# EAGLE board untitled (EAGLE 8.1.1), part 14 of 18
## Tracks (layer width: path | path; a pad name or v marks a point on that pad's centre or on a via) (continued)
S$14098 (continued)
  Bottom 0: 231.52,137.75 231.07,137.79
S$14099
  Bottom 0: 231.07,137.79 230.63,137.75
S$14100
  Bottom 0: 230.63,137.75 230.2,137.62
S$14101
  Bottom 0: 230.2,137.62 229.8,137.41
S$14102
  Bottom 0: 229.8,137.41 229.46,137.12
S$14103
  Bottom 0: 229.46,137.12 229.17,136.78
S$14104
  Bottom 0: 229.17,136.78 228.96,136.38
S$14105
  Bottom 0: 228.96,136.38 228.83,135.96
S$14106
  Bottom 0: 228.83,135.96 228.79,135.51
S$14107
  Bottom 0: 228.79,135.51 228.83,135.06
S$14108
  Bottom 0: 228.83,135.06 228.96,134.63
S$14109
  Bottom 0: 228.96,134.63 229.17,134.24
S$14110
  Bottom 0: 229.17,134.24 229.46,133.89
S$14111
  Bottom 0: 229.46,133.89 229.8,133.61
S$14112
  Bottom 0: 229.8,133.61 230.16,133.42
S$14113
  Bottom 0: 230.16,133.42 225.02,133.42
S$14114
  Bottom 0: 225.02,133.42 215.78,142.65
S$14115
  Bottom 0: 215.78,142.65 216.1,142.67
S$14116
  Bottom 0: 216.1,142.67 216.4,142.78
S$14117
  Bottom 0: 216.4,142.78 216.67,142.97
S$14118
  Bottom 0: 216.67,142.97 216.87,143.22
S$14119
  Bottom 0: 216.87,143.22 217,143.52
S$14120
  Bottom 0: 217,143.52 217.05,143.84
S$14121
  Bottom 0: 217.05,143.84 217,144.16
S$14122
  Bottom 0: 217,144.16 216.87,144.46
S$14123
  Bottom 0: 216.87,144.46 216.67,144.71
S$14124
  Bottom 0: 216.67,144.71 216.4,144.9
S$14125
  Bottom 0: 216.4,144.9 216.1,145.01
S$14126
  Bottom 0: 216.1,145.01 215.77,145.03
S$14127
  Bottom 0: 215.77,145.03 215.45,144.96
S$14128
  Bottom 0: 215.45,144.96 215.16,144.82
S$14129
  Bottom 0: 215.16,144.82 214.93,144.59
S$14130
  Bottom 0: 214.93,144.59 214.76,144.32
S$14131
  Bottom 0: 214.76,144.32 214.67,144
S$14132
  Bottom 0: 214.67,144 214.67,143.77
S$14133
  Bottom 0: 214.67,143.77 199.64,158.8
S$14134
  Bottom 0: 199.64,158.8 199.64,158.84
S$14135
  Bottom 0: 199.64,158.84 199.63,158.91
S$14136
  Bottom 0: 199.63,158.91 199.62,158.98
S$14137
  Bottom 0: 199.62,158.98 199.59,159.04
S$14138
  Bottom 0: 199.59,159.04 199.55,159.1
S$14139
  Bottom 0: 199.55,159.1 199.51,159.16
S$14140
  Bottom 0: 199.51,159.16 198.6,160.06
S$14141
  Bottom 0: 198.6,160.06 198.55,160.1
S$14142
  Bottom 0: 198.55,160.1 198.49,160.14
S$14143
  Bottom 0: 198.49,160.14 198.43,160.17
S$14144
  Bottom 0: 198.43,160.17 198.36,160.18
S$14145
  Bottom 0: 198.36,160.18 198.29,160.19
S$14146
  Bottom 0: 198.29,160.19 197.07,160.19
S$14147
  Bottom 0: 197.07,160.19 197,160.18
S$14148
  Bottom 0: 197,160.18 196.93,160.17
S$14149
  Bottom 0: 196.93,160.17 196.87,160.14
S$14150
  Bottom 0: 196.87,160.14 196.81,160.1
S$14151
  Bottom 0: 196.81,160.1 196.76,160.06
S$14152
  Bottom 0: 196.76,160.06 191.71,155.01
S$14153
  Bottom 0: 191.71,155.01 191.67,154.95
S$14154
  Bottom 0: 191.67,154.95 191.63,154.89
S$14155
  Bottom 0: 191.63,154.89 191.6,154.83
S$14156
  Bottom 0: 191.6,154.83 191.59,154.76
S$14157
  Bottom 0: 191.59,154.76 191.58,154.7
S$14158
  Bottom 0: 191.58,154.7 191.58,153.34
S$14159
  Bottom 0: 191.58,153.34 191.43,153.28
S$14160
  Bottom 0: 191.43,153.28 191.13,153.1
S$14161
  Bottom 0: 191.13,153.1 190.9,152.84
S$14162
  Bottom 0: 190.9,152.84 190.76,152.6
S$14163
  Bottom 0: 190.76,152.6 189.38,152.6
S$14164
  Bottom 0: 189.38,152.6 189.48,152.66
S$14165
  Bottom 0: 189.48,152.66 189.83,152.94
S$14166
  Bottom 0: 189.83,152.94 190.11,153.29
S$14167
  Bottom 0: 190.11,153.29 190.33,153.68
S$14168
  Bottom 0: 190.33,153.68 190.45,154.11
S$14169
  Bottom 0: 190.45,154.11 190.5,154.56
S$14170
  Bottom 0: 190.5,154.56 190.45,155.01
S$14171
  Bottom 0: 190.45,155.01 190.33,155.43
S$14172
  Bottom 0: 190.33,155.43 190.11,155.83
S$14173
  Bottom 0: 190.11,155.83 189.83,156.17
S$14174
  Bottom 0: 189.83,156.17 189.48,156.46
S$14175
  Bottom 0: 189.48,156.46 189.09,156.67
S$14176
  Bottom 0: 189.09,156.67 188.66,156.8
S$14177
  Bottom 0: 188.66,156.8 188.21,156.84
S$14178
  Bottom 0: 188.21,156.84 187.77,156.8
S$14179
  Bottom 0: 187.77,156.8 187.34,156.67
S$14180
  Bottom 0: 187.34,156.67 186.94,156.46
S$14181
  Bottom 0: 186.94,156.46 186.6,156.17
S$14182
  Bottom 0: 186.6,156.17 186.31,155.83
S$14183
  Bottom 0: 186.31,155.83 186.1,155.43
S$14184
  Bottom 0: 186.1,155.43 185.97,155.01
S$14185
  Bottom 0: 185.97,155.01 185.93,154.56
S$14186
  Bottom 0: 185.93,154.56 185.97,154.11
S$14187
  Bottom 0: 185.97,154.11 186.1,153.68
S$14188
  Bottom 0: 186.1,153.68 186.31,153.29
S$14189
  Bottom 0: 186.31,153.29 186.6,152.94
S$14190
  Bottom 0: 186.6,152.94 186.94,152.66
S$14191
  Bottom 0: 186.94,152.66 187.05,152.6
S$14192
  Bottom 0: 187.05,152.6 177.17,152.6
S$14193
  Bottom 0: 177.17,152.6 175.9,153.88
S$14194
  Bottom 0: 175.9,153.88 175.84,153.92
S$14195
  Bottom 0: 175.84,153.92 175.78,153.96
S$14196
  Bottom 0: 175.78,153.96 175.72,153.99
S$14197
  Bottom 0: 175.72,153.99 175.65,154
S$14198
  Bottom 0: 175.65,154 175.58,154
S$14199
  Bottom 0: 175.58,154 171.91,154
S$14200
  Bottom 0: 171.91,154 171.84,154
S$14201
  Bottom 0: 171.84,154 171.77,153.99
S$14202
  Bottom 0: 171.77,153.99 171.71,153.96
S$14203
  Bottom 0: 171.71,153.96 171.65,153.92
S$14204
  Bottom 0: 171.65,153.92 171.59,153.88
S$14205
  Bottom 0: 171.59,153.88 171.13,153.42
S$14206
  Bottom 0: 171.13,153.42 171.28,153.68
S$14207
  Bottom 0: 171.28,153.68 171.4,154.11
S$14208
  Bottom 0: 171.4,154.11 171.45,154.56
S$14209
  Bottom 0: 171.45,154.56 171.4,155.01
S$14210
  Bottom 0: 171.4,155.01 171.28,155.43
S$14211
  Bottom 0: 171.28,155.43 171.06,155.83
S$14212
  Bottom 0: 171.06,155.83 170.78,156.17
S$14213
  Bottom 0: 170.78,156.17 170.43,156.46
S$14214
  Bottom 0: 170.43,156.46 170.04,156.67
S$14215
  Bottom 0: 170.04,156.67 169.61,156.8
S$14216
  Bottom 0: 169.61,156.8 169.16,156.84
S$14217
  Bottom 0: 169.16,156.84 168.72,156.8
S$14218
  Bottom 0: 168.72,156.8 168.29,156.67
S$14219
  Bottom 0: 168.29,156.67 167.89,156.46
S$14220
  Bottom 0: 167.89,156.46 167.55,156.17
S$14221
  Bottom 0: 167.55,156.17 167.26,155.83
S$14222
  Bottom 0: 167.26,155.83 167.05,155.43
S$14223
  Bottom 0: 167.05,155.43 166.92,155.01
S$14224
  Bottom 0: 166.92,155.01 166.88,154.56
S$14225
  Bottom 0: 166.88,154.56 166.92,154.11
S$14226
  Bottom 0: 166.92,154.11 167.05,153.68
S$14227
  Bottom 0: 167.05,153.68 167.26,153.29
S$14228
  Bottom 0: 167.26,153.29 167.55,152.94
S$14229
  Bottom 0: 167.55,152.94 167.89,152.66
S$14230
  Bottom 0: 167.89,152.66 168.08,152.56
S$14231
  Bottom 0: 168.08,152.56 158.57,152.56
S$14232
  Bottom 0: 158.57,152.56 158.57,156.7
S$14233
  Bottom 0: 158.57,156.7 158.56,156.77
S$14234
  Bottom 0: 158.56,156.77 158.55,156.84
S$14235
  Bottom 0: 158.55,156.84 158.52,156.9
S$14236
  Bottom 0: 158.52,156.9 158.48,156.96
S$14237
  Bottom 0: 158.48,156.96 158.44,157.02
S$14238
  Bottom 0: 158.44,157.02 153.73,161.73
S$14239
  Bottom 0: 153.73,161.73 153.86,161.71
S$14240
  Bottom 0: 153.86,161.71 154.18,161.73
S$14241
  Bottom 0: 154.18,161.73 154.49,161.83
S$14242
  Bottom 0: 154.49,161.83 154.75,162.02
S$14243
  Bottom 0: 154.75,162.02 154.96,162.28
S$14244
  Bottom 0: 154.96,162.28 155.09,162.57
S$14245
  Bottom 0: 155.09,162.57 155.13,162.89
S$14246
  Bottom 0: 155.13,162.89 155.09,163.22
S$14247
  Bottom 0: 155.09,163.22 154.96,163.51
S$14248
  Bottom 0: 154.96,163.51 154.75,163.77
S$14249
  Bottom 0: 154.75,163.77 154.49,163.96
S$14250
  Bottom 0: 154.49,163.96 154.18,164.06
S$14251
  Bottom 0: 154.18,164.06 153.86,164.08
S$14252
  Bottom 0: 153.86,164.08 153.54,164.02
S$14253
  Bottom 0: 153.54,164.02 153.25,163.87
S$14254
  Bottom 0: 153.25,163.87 153.01,163.65
S$14255
  Bottom 0: 153.01,163.65 152.84,163.37
S$14256
  Bottom 0: 152.84,163.37 152.76,163.06
S$14257
  Bottom 0: 152.76,163.06 152.76,162.73
S$14258
  Bottom 0: 152.76,162.73 152.77,162.69
S$14259
  Bottom 0: 152.77,162.69 145.38,170.08
S$14260
  Bottom 0: 145.38,170.08 145.41,170.11
S$14261
  Bottom 0: 145.41,170.11 145.62,170.4
S$14262
  Bottom 0: 145.62,170.4 145.75,170.72
S$14263
  Bottom 0: 145.75,170.72 145.8,171.07
S$14264
  Bottom 0: 145.8,171.07 145.75,171.41
S$14265
  Bottom 0: 145.75,171.41 145.62,171.74
S$14266
  Bottom 0: 145.62,171.74 145.41,172.02
S$14267
  Bottom 0: 145.41,172.02 145.15,172.25
S$14268
  Bottom 0: 145.15,172.25 144.83,172.4
S$14269
  Bottom 0: 144.83,172.4 144.49,172.46
S$14270
  Bottom 0: 144.49,172.46 144.13,172.44
S$14271
  Bottom 0: 144.13,172.44 143.81,172.33
S$14272
  Bottom 0: 143.81,172.33 143.51,172.15
S$14273
  Bottom 0: 143.51,172.15 143.27,171.89
S$14274
  Bottom 0: 143.27,171.89 143.1,171.58
S$14275
  Bottom 0: 143.1,171.58 143.01,171.24
S$14276
  Bottom 0: 143.01,171.24 143.01,170.9
S$14277
  Bottom 0: 143.01,170.9 143.1,170.56
S$14278
  Bottom 0: 143.1,170.56 143.27,170.25
S$14279
  Bottom 0: 143.27,170.25 143.51,169.99
S$14280
  Bottom 0: 143.51,169.99 143.81,169.8
S$14281
  Bottom 0: 143.81,169.8 144.13,169.7
S$14282
  Bottom 0: 144.13,169.7 144.49,169.68
S$14283
  Bottom 0: 144.49,169.68 144.52,169.68
S$14284
  Bottom 0: 144.52,169.68 147.18,167.02
S$14285
  Bottom 0: 147.18,167.02 142.66,167.02
S$14286
  Bottom 0: 142.66,167.02 138.47,171.23
S$14287
  Bottom 0: 138.47,171.23 138.47,171.28
S$14288
  Bottom 0: 138.47,171.28 138.43,171.53
S$14289
  Bottom 0: 138.43,171.53 138.3,171.74
S$14290
  Bottom 0: 138.3,171.74 138.09,171.89
S$14291
  Bottom 0: 138.09,171.89 137.85,171.96
S$14292
  Bottom 0: 137.85,171.96 137.6,171.94
S$14293
  Bottom 0: 137.6,171.94 137.38,171.83
S$14294
  Bottom 0: 137.38,171.83 137.2,171.64
S$14295
  Bottom 0: 137.2,171.64 137.11,171.4
S$14296
  Bottom 0: 137.11,171.4 137.11,171.15
S$14297
  Bottom 0: 137.11,171.15 137.2,170.92
S$14298
  Bottom 0: 137.2,170.92 137.38,170.73
S$14299
  Bottom 0: 137.38,170.73 137.6,170.62
S$14300
  Bottom 0: 137.6,170.62 137.85,170.6
S$14301
  Bottom 0: 137.85,170.6 138.67,169.76
S$14302
  Bottom 0: 138.67,169.76 138.48,169.86
S$14303
  Bottom 0: 138.48,169.86 138.13,169.92
S$14304
  Bottom 0: 138.13,169.92 137.78,169.9
S$14305
  Bottom 0: 137.78,169.9 137.46,169.79
S$14306
  Bottom 0: 137.46,169.79 137.16,169.61
S$14307
  Bottom 0: 137.16,169.61 136.92,169.35
S$14308
  Bottom 0: 136.92,169.35 136.8,169.14
S$14309
  Bottom 0: 136.8,169.14 136.8,174.28
S$14310
  Bottom 0: 136.8,174.28 139.63,177.1
S$14311
  Bottom 0: 139.63,177.1 139.66,177.16
S$14312
  Bottom 0: 139.66,177.16 139.7,177.2
S$14313
  Bottom 0: 139.7,177.2 139.71,177.25
S$14314
  Bottom 0: 139.71,177.25 139.74,177.3
S$14315
  Bottom 0: 139.74,177.3 139.74,177.36
S$14316
  Bottom 0: 139.74,177.36 139.76,177.42
S$14317
  Bottom 0: 139.76,177.42 139.76,177.55
S$14318
  Bottom 0: 139.76,177.55 140.21,177.55
S$14319
  Bottom 0: 140.21,177.55 140.28,177.56
S$14320
  Bottom 0: 140.28,177.56 140.35,177.6
S$14321
  Bottom 0: 140.35,177.6 140.41,177.65
S$14322
  Bottom 0: 140.41,177.65 140.45,177.72
S$14323
  Bottom 0: 140.45,177.72 140.46,177.8
S$14324
  Bottom 0: 140.46,177.8 140.46,179.51
S$14325
  Bottom 0: 140.46,179.51 141.07,179.51
S$14326
  Bottom 0: 141.07,179.51 140.9,179.31
S$14327
  Bottom 0: 140.9,179.31 140.76,179.01
S$14328
  Bottom 0: 140.76,179.01 140.72,178.69
S$14329
  Bottom 0: 140.72,178.69 140.76,178.37
S$14330
  Bottom 0: 140.76,178.37 140.9,178.07
S$14331
  Bottom 0: 140.9,178.07 141.11,177.82
S$14332
  Bottom 0: 141.11,177.82 141.39,177.65
S$14333
  Bottom 0: 141.39,177.65 141.7,177.56
S$14334
  Bottom 0: 141.7,177.56 142.02,177.56
S$14335
  Bottom 0: 142.02,177.56 142.33,177.65
S$14336
  Bottom 0: 142.33,177.65 142.61,177.82
S$14337
  Bottom 0: 142.61,177.82 142.82,178.07
S$14338
  Bottom 0: 142.82,178.07 142.96,178.37
S$14339
  Bottom 0: 142.96,178.37 143,178.69
S$14340
  Bottom 0: 143,178.69 142.96,179.01
S$14341
  Bottom 0: 142.96,179.01 142.82,179.31
S$14342
  Bottom 0: 142.82,179.31 142.65,179.51
S$14343
  Bottom 0: 142.65,179.51 157.23,179.51
S$14344
  Bottom 0: 157.23,179.51 157.23,177.8
S$14345
  Bottom 0: 157.23,177.8 157.24,177.72
S$14346
  Bottom 0: 157.24,177.72 157.28,177.65
S$14347
  Bottom 0: 157.28,177.65 157.33,177.6
S$14348
  Bottom 0: 157.33,177.6 157.4,177.56
S$14349
  Bottom 0: 157.4,177.56 157.48,177.55
S$14350
  Bottom 0: 157.48,177.55 157.87,177.55
S$14351
  Bottom 0: 157.87,177.55 155.15,174.83
S$14352
  Bottom 0: 155.15,174.83 155.1,174.77
S$14353
  Bottom 0: 155.1,174.77 155.07,174.72
S$14354
  Bottom 0: 155.07,174.72 155.04,174.65
S$14355
  Bottom 0: 155.04,174.65 155.02,174.58
S$14356
  Bottom 0: 155.02,174.58 155.01,174.51
S$14357
  Bottom 0: 155.01,174.51 155.01,166.12
S$14358
  Bottom 0: 155.01,166.12 154.92,166.03
S$14359
  Bottom 0: 154.92,166.03 154.75,165.75
S$14360
  Bottom 0: 154.75,165.75 154.66,165.43
S$14361
  Bottom 0: 154.66,165.43 154.66,165.11
S$14362
  Bottom 0: 154.66,165.11 154.75,164.79
S$14363
  Bottom 0: 154.75,164.79 154.92,164.52
S$14364
  Bottom 0: 154.92,164.52 155.15,164.3
S$14365
  Bottom 0: 155.15,164.3 155.44,164.15
S$14366
  Bottom 0: 155.44,164.15 155.76,164.08
S$14367
  Bottom 0: 155.76,164.08 156.09,164.1
S$14368
  Bottom 0: 156.09,164.1 156.39,164.21
S$14369
  Bottom 0: 156.39,164.21 156.66,164.4
S$14370
  Bottom 0: 156.66,164.4 156.87,164.65
S$14371
  Bottom 0: 156.87,164.65 156.99,164.95
S$14372
  Bottom 0: 156.99,164.95 157.04,165.27
S$14373
  Bottom 0: 157.04,165.27 156.99,165.59
S$14374
  Bottom 0: 156.99,165.59 156.87,165.89
S$14375
  Bottom 0: 156.87,165.89 156.66,166.15
S$14376
  Bottom 0: 156.66,166.15 156.39,166.33
S$14377
  Bottom 0: 156.39,166.33 156.09,166.44
S$14378
  Bottom 0: 156.09,166.44 155.9,166.45
S$14379
  Bottom 0: 155.9,166.45 155.9,167.83
S$14380
  Bottom 0: 155.9,167.83 155.97,167.71
S$14381
  Bottom 0: 155.97,167.71 156.21,167.45
S$14382
  Bottom 0: 156.21,167.45 156.5,167.26
S$14383
  Bottom 0: 156.5,167.26 156.84,167.16
S$14384
  Bottom 0: 156.84,167.16 157.19,167.14
S$14385
  Bottom 0: 157.19,167.14 157.53,167.2
S$14386
  Bottom 0: 157.53,167.2 157.85,167.35
S$14387
  Bottom 0: 157.85,167.35 158.12,167.57
S$14388
  Bottom 0: 158.12,167.57 158.32,167.86
S$14389
  Bottom 0: 158.32,167.86 158.45,168.18
S$14390
  Bottom 0: 158.45,168.18 158.5,168.53
S$14391
  Bottom 0: 158.5,168.53 158.45,168.87
S$14392
  Bottom 0: 158.45,168.87 158.32,169.2
S$14393
  Bottom 0: 158.32,169.2 158.12,169.48
S$14394
  Bottom 0: 158.12,169.48 157.85,169.71
S$14395
  Bottom 0: 157.85,169.71 157.53,169.86
S$14396
  Bottom 0: 157.53,169.86 157.19,169.92
S$14397
  Bottom 0: 157.19,169.92 156.84,169.9
S$14398
  Bottom 0: 156.84,169.9 156.5,169.79
S$14399
  Bottom 0: 156.5,169.79 156.21,169.61
S$14400
  Bottom 0: 156.21,169.61 155.97,169.35
S$14401
  Bottom 0: 155.97,169.35 155.9,169.22
S$14402
  Bottom 0: 155.9,169.22 155.9,174.33
S$14403
  Bottom 0: 155.9,174.33 158.68,177.1
S$14404
  Bottom 0: 158.68,177.1 158.71,177.16
S$14405
  Bottom 0: 158.71,177.16 158.75,177.2
S$14406
  Bottom 0: 158.75,177.2 158.76,177.25
S$14407
  Bottom 0: 158.76,177.25 158.79,177.3
S$14408
  Bottom 0: 158.79,177.3 158.79,177.36
S$14409
  Bottom 0: 158.79,177.36 158.81,177.42
S$14410
  Bottom 0: 158.81,177.42 158.81,177.55
S$14411
  Bottom 0: 158.81,177.55 159.26,177.55
S$14412
  Bottom 0: 159.26,177.55 159.33,177.56
S$14413
  Bottom 0: 159.33,177.56 159.41,177.6
S$14414
  Bottom 0: 159.41,177.6 159.46,177.65
S$14415
  Bottom 0: 159.46,177.65 159.5,177.72
S$14416
  Bottom 0: 159.5,177.72 159.51,177.8
S$14417
  Bottom 0: 159.51,177.8 159.51,179.51
S$14418
  Bottom 0: 159.51,179.51 160.12,179.51
S$14419
  Bottom 0: 160.12,179.51 159.95,179.31
S$14420
  Bottom 0: 159.95,179.31 159.81,179.01
S$14421
  Bottom 0: 159.81,179.01 159.77,178.69
S$14422
  Bottom 0: 159.77,178.69 159.81,178.37
S$14423
  Bottom 0: 159.81,178.37 159.95,178.07
S$14424
  Bottom 0: 159.95,178.07 160.16,177.82
S$14425
  Bottom 0: 160.16,177.82 160.44,177.65
S$14426
  Bottom 0: 160.44,177.65 160.75,177.56
S$14427
  Bottom 0: 160.75,177.56 161.07,177.56
S$14428
  Bottom 0: 161.07,177.56 161.2,177.6
S$14429
  Bottom 0: 161.2,177.6 161.59,177.2
S$14430
  Bottom 0: 161.59,177.2 161.59,174.78
S$14431
  Bottom 0: 161.59,174.78 161.54,174.88
S$14432
  Bottom 0: 161.54,174.88 161.25,175.22
S$14433
  Bottom 0: 161.25,175.22 160.91,175.51
S$14434
  Bottom 0: 160.91,175.51 160.51,175.72
S$14435
  Bottom 0: 160.51,175.72 160.09,175.85
S$14436
  Bottom 0: 160.09,175.85 159.64,175.9
S$14437
  Bottom 0: 159.64,175.9 159.19,175.85
S$14438
  Bottom 0: 159.19,175.85 158.76,175.72
S$14439
  Bottom 0: 158.76,175.72 158.37,175.51
S$14440
  Bottom 0: 158.37,175.51 158.02,175.22
S$14441
  Bottom 0: 158.02,175.22 157.74,174.88
S$14442
  Bottom 0: 157.74,174.88 157.52,174.48
S$14443
  Bottom 0: 157.52,174.48 157.4,174.06
S$14444
  Bottom 0: 157.4,174.06 157.35,173.61
S$14445
  Bottom 0: 157.35,173.61 157.4,173.16
S$14446
  Bottom 0: 157.4,173.16 157.52,172.74
S$14447
  Bottom 0: 157.52,172.74 157.74,172.34
S$14448
  Bottom 0: 157.74,172.34 158.02,171.99
S$14449
  Bottom 0: 158.02,171.99 158.37,171.71
S$14450
  Bottom 0: 158.37,171.71 158.76,171.5
S$14451
  Bottom 0: 158.76,171.5 159.19,171.37
S$14452
  Bottom 0: 159.19,171.37 159.64,171.32
S$14453
  Bottom 0: 159.64,171.32 160.09,171.37
S$14454
  Bottom 0: 160.09,171.37 160.51,171.5
S$14455
  Bottom 0: 160.51,171.5 160.91,171.71
S$14456
  Bottom 0: 160.91,171.71 161.11,171.87
S$14457
  Bottom 0: 161.11,171.87 161.11,163.22
S$14458
  Bottom 0: 161.11,163.22 161.11,163.12
S$14459
  Bottom 0: 161.11,163.12 161.13,163.04
S$14460
  Bottom 0: 161.13,163.04 161.17,162.95
S$14461
  Bottom 0: 161.17,162.95 161.21,162.88
S$14462
  Bottom 0: 161.21,162.88 161.28,162.81
S$14463
  Bottom 0: 161.28,162.81 166.24,157.85
S$14464
  Bottom 0: 166.24,157.85 166.3,157.79
S$14465
  Bottom 0: 166.3,157.79 166.38,157.74
S$14466
  Bottom 0: 166.38,157.74 166.46,157.71
S$14467
  Bottom 0: 166.46,157.71 166.55,157.69
S$14468
  Bottom 0: 166.55,157.69 166.64,157.68
S$14469
  Bottom 0: 166.64,157.68 169.05,157.68
S$14470
  Bottom 0: 169.05,157.68 169.14,157.69
S$14471
  Bottom 0: 169.14,157.69 169.22,157.71
S$14472
  Bottom 0: 169.22,157.71 169.31,157.74
S$14473
  Bottom 0: 169.31,157.74 169.38,157.79
S$14474
  Bottom 0: 169.38,157.79 169.45,157.85
S$14475
  Bottom 0: 169.45,157.85 170.14,158.55
S$14476
  Bottom 0: 170.14,158.55 170.27,158.51
S$14477
  Bottom 0: 170.27,158.51 170.6,158.51
S$14478
  Bottom 0: 170.6,158.51 170.9,158.6
S$14479
  Bottom 0: 170.9,158.6 171.18,158.78
S$14480
  Bottom 0: 171.18,158.78 171.39,159.02
S$14481
  Bottom 0: 171.39,159.02 171.53,159.32
S$14482
  Bottom 0: 171.53,159.32 171.58,159.64
S$14483
  Bottom 0: 171.58,159.64 171.53,159.96
S$14484
  Bottom 0: 171.53,159.96 171.39,160.26
S$14485
  Bottom 0: 171.39,160.26 171.18,160.5
S$14486
  Bottom 0: 171.18,160.5 170.9,160.68
S$14487
  Bottom 0: 170.9,160.68 170.6,160.77
S$14488
  Bottom 0: 170.6,160.77 170.27,160.77
S$14489
  Bottom 0: 170.27,160.77 169.96,160.68
S$14490
  Bottom 0: 169.96,160.68 169.69,160.5
S$14491
  Bottom 0: 169.69,160.5 169.47,160.26
S$14492
  Bottom 0: 169.47,160.26 169.34,159.96
S$14493
  Bottom 0: 169.34,159.96 169.29,159.64
S$14494
  Bottom 0: 169.29,159.64 169.33,159.34
S$14495
  Bottom 0: 169.33,159.34 169.04,159.04
S$14496
  Bottom 0: 169.04,159.04 169.04,160.53
S$14497
  Bottom 0: 169.04,160.53 169.03,160.6
S$14498
  Bottom 0: 169.03,160.6 168.99,160.68
S$14499
  Bottom 0: 168.99,160.68 168.93,160.73
S$14500
  Bottom 0: 168.93,160.73 168.86,160.77
S$14501
  Bottom 0: 168.86,160.77 168.78,160.78
S$14502
  Bottom 0: 168.78,160.78 168.34,160.78
S$14503
  Bottom 0: 168.34,160.78 168.34,160.91
S$14504
  Bottom 0: 168.34,160.91 168.28,161.13
S$14505
  Bottom 0: 168.28,161.13 168.11,161.29
S$14506
  Bottom 0: 168.11,161.29 167.89,161.35
S$14507
  Bottom 0: 167.89,161.35 167.54,161.35
S$14508
  Bottom 0: 167.54,161.35 166.45,162.43
S$14509
  Bottom 0: 166.45,162.43 166.52,162.57
S$14510
  Bottom 0: 166.52,162.57 166.56,162.89
S$14511
  Bottom 0: 166.56,162.89 166.52,163.22
S$14512
  Bottom 0: 166.52,163.22 166.39,163.51
S$14513
  Bottom 0: 166.39,163.51 166.18,163.77
S$14514
  Bottom 0: 166.18,163.77 165.92,163.96
S$14515
  Bottom 0: 165.92,163.96 165.61,164.06
S$14516
  Bottom 0: 165.61,164.06 165.29,164.08
S$14517
  Bottom 0: 165.29,164.08 164.97,164.02
S$14518
  Bottom 0: 164.97,164.02 164.68,163.87
S$14519
  Bottom 0: 164.68,163.87 164.44,163.65
S$14520
  Bottom 0: 164.44,163.65 164.27,163.37
S$14521
  Bottom 0: 164.27,163.37 164.19,163.06
S$14522
  Bottom 0: 164.19,163.06 164.19,162.73
S$14523
  Bottom 0: 164.19,162.73 164.27,162.42
S$14524
  Bottom 0: 164.27,162.42 164.44,162.14
S$14525
  Bottom 0: 164.44,162.14 164.68,161.92
S$14526
  Bottom 0: 164.68,161.92 164.97,161.77
S$14527
  Bottom 0: 164.97,161.77 165.29,161.71
S$14528
  Bottom 0: 165.29,161.71 165.61,161.73
S$14529
  Bottom 0: 165.61,161.73 165.84,161.8
S$14530
  Bottom 0: 165.84,161.8 166.89,160.75
S$14531
  Bottom 0: 166.89,160.75 166.86,160.73
S$14532
  Bottom 0: 166.86,160.73 166.8,160.68
S$14533
  Bottom 0: 166.8,160.68 166.76,160.6
S$14534
  Bottom 0: 166.76,160.6 166.75,160.53
S$14535
  Bottom 0: 166.75,160.53 166.75,158.94
S$14536
  Bottom 0: 166.75,158.94 162.25,163.45
S$14537
  Bottom 0: 162.25,163.45 162.25,170.38
S$14538
  Bottom 0: 162.25,170.38 162.32,170.25
S$14539
  Bottom 0: 162.32,170.25 162.56,169.99
S$14540
  Bottom 0: 162.56,169.99 162.85,169.8
S$14541
  Bottom 0: 162.85,169.8 163.19,169.7
S$14542
  Bottom 0: 163.19,169.7 163.53,169.68
S$14543
  Bottom 0: 163.53,169.68 163.88,169.74
S$14544
  Bottom 0: 163.88,169.74 164.06,169.82
S$14545
  Bottom 0: 164.06,169.82 167.43,166.46
S$14546
  Bottom 0: 167.43,166.46 167.49,166.42
S$14547
  Bottom 0: 167.49,166.42 167.55,166.38
S$14548
  Bottom 0: 167.55,166.38 167.61,166.35
S$14549
  Bottom 0: 167.61,166.35 167.68,166.33
S$14550
  Bottom 0: 167.68,166.33 167.75,166.33
S$14551
  Bottom 0: 167.75,166.33 171.33,166.33
S$14552
  Bottom 0: 171.33,166.33 174.01,163.64
S$14553
  Bottom 0: 174.01,163.64 174.07,163.6
S$14554
  Bottom 0: 174.07,163.6 174.13,163.56
S$14555
  Bottom 0: 174.13,163.56 174.19,163.53
S$14556
  Bottom 0: 174.19,163.53 174.26,163.52
S$14557
  Bottom 0: 174.26,163.52 174.33,163.51
S$14558
  Bottom 0: 174.33,163.51 178.12,163.51
S$14559
  Bottom 0: 178.12,163.51 178.19,163.52
S$14560
  Bottom 0: 178.19,163.52 178.25,163.53
S$14561
  Bottom 0: 178.25,163.53 178.31,163.56
S$14562
  Bottom 0: 178.31,163.56 178.37,163.6
S$14563
  Bottom 0: 178.37,163.6 178.43,163.64
S$14564
  Bottom 0: 178.43,163.64 180.96,166.17
S$14565
  Bottom 0: 180.96,166.17 181.75,166.17
S$14566
  Bottom 0: 181.75,166.17 181.59,166.02
S$14567
  Bottom 0: 181.59,166.02 181.42,165.75
S$14568
  Bottom 0: 181.42,165.75 181.34,165.43
S$14569
  Bottom 0: 181.34,165.43 181.34,165.1
S$14570
  Bottom 0: 181.34,165.1 181.38,164.93
S$14571
  Bottom 0: 181.38,164.93 179.91,163.46
S$14572
  Bottom 0: 179.91,163.46 174.03,163.46
S$14573
  Bottom 0: 174.03,163.46 174.01,163.51
S$14574
  Bottom 0: 174.01,163.51 173.8,163.77
S$14575
  Bottom 0: 173.8,163.77 173.54,163.96
S$14576
  Bottom 0: 173.54,163.96 173.23,164.06
S$14577
  Bottom 0: 173.23,164.06 172.91,164.08
S$14578
  Bottom 0: 172.91,164.08 172.66,164.03
S$14579
  Bottom 0: 172.66,164.03 171.02,165.67
S$14580
  Bottom 0: 171.02,165.67 170.95,165.74
S$14581
  Bottom 0: 170.95,165.74 170.88,165.78
S$14582
  Bottom 0: 170.88,165.78 170.79,165.81
S$14583
  Bottom 0: 170.79,165.81 170.71,165.84
S$14584
  Bottom 0: 170.71,165.84 170.62,165.84
S$14585
  Bottom 0: 170.62,165.84 164.51,165.84
S$14586
  Bottom 0: 164.51,165.84 164.49,165.89
S$14587
  Bottom 0: 164.49,165.89 164.28,166.15
S$14588
  Bottom 0: 164.28,166.15 164.01,166.33
S$14589
  Bottom 0: 164.01,166.33 163.71,166.44
S$14590
  Bottom 0: 163.71,166.44 163.38,166.46
S$14591
  Bottom 0: 163.38,166.46 163.06,166.4
S$14592
  Bottom 0: 163.06,166.4 162.77,166.25
S$14593
  Bottom 0: 162.77,166.25 162.54,166.03
S$14594
  Bottom 0: 162.54,166.03 162.37,165.75
S$14595
  Bottom 0: 162.37,165.75 162.28,165.43
S$14596
  Bottom 0: 162.28,165.43 162.28,165.11
S$14597
  Bottom 0: 162.28,165.11 162.37,164.79
S$14598
  Bottom 0: 162.37,164.79 162.54,164.52
S$14599
  Bottom 0: 162.54,164.52 162.77,164.3
S$14600
  Bottom 0: 162.77,164.3 163.06,164.15
S$14601
  Bottom 0: 163.06,164.15 163.38,164.08
S$14602
  Bottom 0: 163.38,164.08 163.71,164.1
S$14603
  Bottom 0: 163.71,164.1 164.01,164.21
S$14604
  Bottom 0: 164.01,164.21 164.28,164.4
S$14605
  Bottom 0: 164.28,164.4 164.49,164.65
S$14606
  Bottom 0: 164.49,164.65 164.51,164.7
S$14607
  Bottom 0: 164.51,164.7 170.38,164.7
S$14608
  Bottom 0: 170.38,164.7 171.85,163.23
S$14609
  Bottom 0: 171.85,163.23 171.81,163.06
S$14610
  Bottom 0: 171.81,163.06 171.81,162.73
S$14611
  Bottom 0: 171.81,162.73 171.89,162.42
S$14612
  Bottom 0: 171.89,162.42 172.06,162.14
S$14613
  Bottom 0: 172.06,162.14 172.3,161.92
S$14614
  Bottom 0: 172.3,161.92 172.59,161.77
S$14615
  Bottom 0: 172.59,161.77 172.91,161.71
S$14616
  Bottom 0: 172.91,161.71 173.23,161.73
S$14617
  Bottom 0: 173.23,161.73 173.54,161.83
S$14618
  Bottom 0: 173.54,161.83 173.8,162.02
S$14619
  Bottom 0: 173.8,162.02 174.01,162.28
S$14620
  Bottom 0: 174.01,162.28 174.03,162.33
S$14621
  Bottom 0: 174.03,162.33 180.15,162.33
S$14622
  Bottom 0: 180.15,162.33 180.24,162.33
S$14623
  Bottom 0: 180.24,162.33 180.32,162.35
S$14624
  Bottom 0: 180.32,162.35 180.41,162.38
S$14625
  Bottom 0: 180.41,162.38 180.48,162.43
S$14626
  Bottom 0: 180.48,162.43 180.55,162.49
S$14627
  Bottom 0: 180.55,162.49 182.18,164.13
S$14628
  Bottom 0: 182.18,164.13 182.44,164.08
S$14629
  Bottom 0: 182.44,164.08 182.76,164.1
S$14630
  Bottom 0: 182.76,164.1 183.07,164.21
S$14631
  Bottom 0: 183.07,164.21 183.33,164.39
S$14632
  Bottom 0: 183.33,164.39 183.54,164.65
S$14633
  Bottom 0: 183.54,164.65 183.56,164.7
S$14634
  Bottom 0: 183.56,164.7 189.44,164.7
S$14635
  Bottom 0: 189.44,164.7 190.9,163.23
S$14636
  Bottom 0: 190.9,163.23 190.86,163.06
S$14637
  Bottom 0: 190.86,163.06 190.86,162.73
S$14638
  Bottom 0: 190.86,162.73 190.95,162.42
S$14639
  Bottom 0: 190.95,162.42 191.12,162.14
S$14640
  Bottom 0: 191.12,162.14 191.35,161.92
S$14641
  Bottom 0: 191.35,161.92 191.64,161.77
S$14642
  Bottom 0: 191.64,161.77 191.96,161.71
S$14643
  Bottom 0: 191.96,161.71 192.29,161.73
S$14644
  Bottom 0: 192.29,161.73 192.59,161.83
S$14645
  Bottom 0: 192.59,161.83 192.86,162.02
S$14646
  Bottom 0: 192.86,162.02 193.06,162.28
S$14647
  Bottom 0: 193.06,162.28 193.19,162.57
S$14648
  Bottom 0: 193.19,162.57 193.24,162.89
S$14649
  Bottom 0: 193.24,162.89 193.2,163.14
S$14650
  Bottom 0: 193.2,163.14 194.08,162.26
S$14651
  Bottom 0: 194.08,162.26 194.14,162.22
S$14652
  Bottom 0: 194.14,162.22 194.2,162.18
S$14653
  Bottom 0: 194.2,162.18 194.26,162.15
S$14654
  Bottom 0: 194.26,162.15 194.32,162.14
S$14655
  Bottom 0: 194.32,162.14 194.39,162.13
S$14656
  Bottom 0: 194.39,162.13 199.71,162.13
S$14657
  Bottom 0: 199.71,162.13 204.44,157.4
S$14658
  Bottom 0: 204.44,157.4 204.49,157.36
S$14659
  Bottom 0: 204.49,157.36 204.55,157.32
S$14660
  Bottom 0: 204.55,157.32 204.62,157.3
S$14661
  Bottom 0: 204.62,157.3 204.68,157.28
S$14662
  Bottom 0: 204.68,157.28 204.75,157.28
S$14663
  Bottom 0: 204.75,157.28 207.31,157.28
S$14664
  Bottom 0: 207.31,157.28 207.82,156.77
S$14665
  Bottom 0: 207.82,156.77 207.71,156.8
S$14666
  Bottom 0: 207.71,156.8 207.26,156.84
S$14667
  Bottom 0: 207.26,156.84 206.82,156.8
S$14668
  Bottom 0: 206.82,156.8 206.39,156.67
S$14669
  Bottom 0: 206.39,156.67 205.99,156.46
S$14670
  Bottom 0: 205.99,156.46 205.65,156.17
S$14671
  Bottom 0: 205.65,156.17 205.36,155.83
S$14672
  Bottom 0: 205.36,155.83 205.15,155.43
S$14673
  Bottom 0: 205.15,155.43 205.02,155.01
S$14674
  Bottom 0: 205.02,155.01 204.98,154.56
S$14675
  Bottom 0: 204.98,154.56 205.02,154.11
S$14676
  Bottom 0: 205.02,154.11 205.15,153.68
S$14677
  Bottom 0: 205.15,153.68 205.36,153.29
S$14678
  Bottom 0: 205.36,153.29 205.65,152.94
S$14679
  Bottom 0: 205.65,152.94 205.99,152.66
S$14680
  Bottom 0: 205.99,152.66 206.39,152.45
S$14681
  Bottom 0: 206.39,152.45 206.82,152.32
S$14682
  Bottom 0: 206.82,152.32 207.26,152.27
S$14683
  Bottom 0: 207.26,152.27 207.71,152.32
S$14684
  Bottom 0: 207.71,152.32 208.14,152.45
S$14685
  Bottom 0: 208.14,152.45 208.53,152.66
S$14686
  Bottom 0: 208.53,152.66 208.88,152.94
S$14687
  Bottom 0: 208.88,152.94 209.16,153.29
S$14688
  Bottom 0: 209.16,153.29 209.38,153.68
S$14689
  Bottom 0: 209.38,153.68 209.5,154.11
S$14690
  Bottom 0: 209.5,154.11 209.55,154.56
S$14691
  Bottom 0: 209.55,154.56 209.5,155.01
S$14692
  Bottom 0: 209.5,155.01 209.47,155.11
S$14693
  Bottom 0: 209.47,155.11 211.18,153.41
S$14694
  Bottom 0: 211.18,153.41 211.16,153.41
S$14695
  Bottom 0: 211.16,153.41 210.81,153.39
S$14696
  Bottom 0: 210.81,153.39 210.48,153.28
S$14697
  Bottom 0: 210.48,153.28 210.19,153.1
S$14698
  Bottom 0: 210.19,153.1 209.95,152.84
S$14699
  Bottom 0: 209.95,152.84 209.77,152.53
S$14700
  Bottom 0: 209.77,152.53 209.69,152.19
S$14701
  Bottom 0: 209.69,152.19 209.69,151.84
S$14702
  Bottom 0: 209.69,151.84 209.77,151.51
S$14703
  Bottom 0: 209.77,151.51 209.95,151.2
S$14704
  Bottom 0: 209.95,151.2 210.19,150.94
S$14705
  Bottom 0: 210.19,150.94 210.48,150.75
S$14706
  Bottom 0: 210.48,150.75 210.81,150.65
S$14707
  Bottom 0: 210.81,150.65 211.16,150.63
S$14708
  Bottom 0: 211.16,150.63 211.51,150.69
S$14709
  Bottom 0: 211.51,150.69 211.82,150.84
S$14710
  Bottom 0: 211.82,150.84 212.09,151.06
S$14711
  Bottom 0: 212.09,151.06 212.3,151.35
S$14712
  Bottom 0: 212.3,151.35 212.43,151.67
S$14713
  Bottom 0: 212.43,151.67 212.47,152.02
S$14714
  Bottom 0: 212.47,152.02 212.46,152.13
S$14715
  Bottom 0: 212.46,152.13 223.05,141.53
S$14716
  Bottom 0: 223.05,141.53 223.11,141.49
S$14717
  Bottom 0: 223.11,141.49 223.17,141.45
S$14718
  Bottom 0: 223.17,141.45 223.23,141.43
S$14719
  Bottom 0: 223.23,141.43 223.29,141.41
S$14720
  Bottom 0: 223.29,141.41 223.37,141.41
S$14721
  Bottom 0: 223.37,141.41 228.66,141.41
S$14722
  Bottom 0: 228.66,141.41 228.66,139.69
S$14723
  Bottom 0: 228.66,139.69 222.56,139.69
S$14724
  Bottom 0: 222.56,139.69 222.54,139.85
S$14725
  Bottom 0: 222.54,139.85 222.41,140.13
S$14726
  Bottom 0: 222.41,140.13 222.2,140.34
S$14727
  Bottom 0: 222.2,140.34 221.94,140.5
S$14728
  Bottom 0: 221.94,140.5 221.64,140.56
S$14729
  Bottom 0: 221.64,140.56 221.34,140.54
S$14730
  Bottom 0: 221.34,140.54 221.06,140.43
S$14731
  Bottom 0: 221.06,140.43 220.82,140.24
S$14732
  Bottom 0: 220.82,140.24 220.66,140
S$14733
  Bottom 0: 220.66,140 220.56,139.71
S$14734
  Bottom 0: 220.56,139.71 220.56,139.4
S$14735
  Bottom 0: 220.56,139.4 220.66,139.11
S$14736
  Bottom 0: 220.66,139.11 220.82,138.86
S$14737
  Bottom 0: 220.82,138.86 221.06,138.67
S$14738
  Bottom 0: 221.06,138.67 221.34,138.56
S$14739
  Bottom 0: 221.34,138.56 221.64,138.54
S$14740
  Bottom 0: 221.64,138.54 221.94,138.61
S$14741
  Bottom 0: 221.94,138.61 222.2,138.76
S$14742
  Bottom 0: 222.2,138.76 222.25,138.81
S$14743
  Bottom 0: 222.25,138.81 239.95,138.81
S$14744
  Bottom 0: 239.95,138.81 240.11,138.67
S$14745
  Bottom 0: 240.11,138.67 240.4,138.56
S$14746
  Bottom 0: 240.4,138.56 240.7,138.54
S$14747
  Bottom 0: 240.7,138.54 241,138.61
S$14748
  Bottom 0: 241,138.61 241.26,138.76
S$14749
  Bottom 0: 241.26,138.76 241.46,138.98
S$14750
  Bottom 0: 241.46,138.98 241.59,139.25
S$14751
  Bottom 0: 241.59,139.25 241.64,139.55
S$14752
  Bottom 0: 241.64,139.55 241.59,139.85
S$14753
  Bottom 0: 241.59,139.85 241.46,140.13
S$14754
  Bottom 0: 241.46,140.13 241.26,140.34
S$14755
  Bottom 0: 241.26,140.34 241,140.5
S$14756
  Bottom 0: 241,140.5 240.7,140.56
S$14757
  Bottom 0: 240.7,140.56 240.4,140.54
S$14758
  Bottom 0: 240.4,140.54 240.11,140.43
S$14759
  Bottom 0: 240.11,140.43 239.88,140.24
S$14760
  Bottom 0: 239.88,140.24 239.71,140
S$14761
  Bottom 0: 239.71,140 239.62,139.71
S$14762
  Bottom 0: 239.62,139.71 239.62,139.69
S$14763
  Bottom 0: 239.62,139.69 233.03,139.69
S$14764
  Bottom 0: 233.03,139.69 233.09,139.72
S$14765
  Bottom 0: 233.09,139.72 233.3,139.97
S$14766
  Bottom 0: 233.3,139.97 233.44,140.27
S$14767
  Bottom 0: 233.44,140.27 233.49,140.59
S$14768
  Bottom 0: 233.49,140.59 233.44,140.91
S$14769
  Bottom 0: 233.44,140.91 233.3,141.21
S$14770
  Bottom 0: 233.3,141.21 233.13,141.41
S$14771
  Bottom 0: 233.13,141.41 240.46,141.41
S$14772
  Bottom 0: 240.46,141.41 242.17,139.69
S$14773
  Bottom 0: 242.17,139.69 242.17,139.52
S$14774
  Bottom 0: 242.17,139.52 242.22,139.39
S$14775
  Bottom 0: 242.22,139.39 242.11,139.38
S$14776
  Bottom 0: 242.11,139.38 241.89,139.27
S$14777
  Bottom 0: 241.89,139.27 241.72,139.08
S$14778
  Bottom 0: 241.72,139.08 241.62,138.85
S$14779
  Bottom 0: 241.62,138.85 241.62,138.59
S$14780
  Bottom 0: 241.62,138.59 241.72,138.36
S$14781
  Bottom 0: 241.72,138.36 241.76,138.31
S$14782
  Bottom 0: 241.76,138.31 236.26,132.82
S$14783
  Bottom 0: 178.78,157.59 179.07,157.66
S$14784
  Bottom 0: 179.07,157.66 179.34,157.81
S$14785
  Bottom 0: 179.34,157.81 179.54,158.03
S$14786
  Bottom 0: 179.54,158.03 179.68,158.3
S$14787
  Bottom 0: 179.68,158.3 179.72,158.6
S$14788
  Bottom 0: 179.72,158.6 179.68,158.9
S$14789
  Bottom 0: 179.68,158.9 179.54,159.18
S$14790
  Bottom 0: 179.54,159.18 179.34,159.4
S$14791
  Bottom 0: 179.34,159.4 179.07,159.55
S$14792
  Bottom 0: 179.07,159.55 178.78,159.61
S$14793
  Bottom 0: 178.78,159.61 178.48,159.59
S$14794
  Bottom 0: 178.48,159.59 178.2,159.48
S$14795
  Bottom 0: 178.2,159.48 177.96,159.29
S$14796
  Bottom 0: 177.96,159.29 177.79,159.04
S$14797
  Bottom 0: 177.79,159.04 177.7,158.75
S$14798
  Bottom 0: 177.7,158.75 177.7,158.45
S$14799
  Bottom 0: 177.7,158.45 177.79,158.16
S$14800
  Bottom 0: 177.79,158.16 177.96,157.91
S$14801
  Bottom 0: 177.96,157.91 178.2,157.72
S$14802
  Bottom 0: 178.2,157.72 178.48,157.61
S$14803
  Bottom 0: 178.48,157.61 178.78,157.59
S$14804
  Bottom 0: 159.73,157.59 160.03,157.66
S$14805
  Bottom 0: 160.03,157.66 160.29,157.81
S$14806
  Bottom 0: 160.29,157.81 160.49,158.03
S$14807
  Bottom 0: 160.49,158.03 160.62,158.3
S$14808
  Bottom 0: 160.62,158.3 160.67,158.6
S$14809
  Bottom 0: 160.67,158.6 160.62,158.9
S$14810
  Bottom 0: 160.62,158.9 160.49,159.18
S$14811
  Bottom 0: 160.49,159.18 160.29,159.4
S$14812
  Bottom 0: 160.29,159.4 160.03,159.55
S$14813
  Bottom 0: 160.03,159.55 159.73,159.61
S$14814
  Bottom 0: 159.73,159.61 159.43,159.59
S$14815
  Bottom 0: 159.43,159.59 159.14,159.48
S$14816
  Bottom 0: 159.14,159.48 158.91,159.29
S$14817
  Bottom 0: 158.91,159.29 158.74,159.04
S$14818
  Bottom 0: 158.74,159.04 158.65,158.75
S$14819
  Bottom 0: 158.65,158.75 158.65,158.45
S$14820
  Bottom 0: 158.65,158.45 158.74,158.16
S$14821
  Bottom 0: 158.74,158.16 158.91,157.91
S$14822
  Bottom 0: 158.91,157.91 159.14,157.72
S$14823
  Bottom 0: 159.14,157.72 159.43,157.61
S$14824
  Bottom 0: 159.43,157.61 159.73,157.59
S$14825
  Bottom 0: 186.06,158.5 187.83,158.5
S$14826
  Bottom 0: 187.83,158.5 187.91,158.51
S$14827
  Bottom 0: 187.91,158.51 187.98,158.55
S$14828
  Bottom 0: 187.98,158.55 188.04,158.6
S$14829
  Bottom 0: 188.04,158.6 188.08,158.67
S$14830
  Bottom 0: 188.08,158.67 188.09,158.75
S$14831
  Bottom 0: 188.09,158.75 188.09,160.53
S$14832
  Bottom 0: 188.09,160.53 188.08,160.6
S$14833
  Bottom 0: 188.08,160.6 188.04,160.68
S$14834
  Bottom 0: 188.04,160.68 187.98,160.73
S$14835
  Bottom 0: 187.98,160.73 187.91,160.77
S$14836
  Bottom 0: 187.91,160.77 187.83,160.78
S$14837
  Bottom 0: 187.83,160.78 187.39,160.78
S$14838
  Bottom 0: 187.39,160.78 187.39,160.91
S$14839
  Bottom 0: 187.39,160.91 187.32,161.13
S$14840
  Bottom 0: 187.32,161.13 187.16,161.29
S$14841
  Bottom 0: 187.16,161.29 186.94,161.35
S$14842
  Bottom 0: 186.94,161.35 186.6,161.35
S$14843
  Bottom 0: 186.6,161.35 185.51,162.44
S$14844
  Bottom 0: 185.51,162.44 185.57,162.57
S$14845
  Bottom 0: 185.57,162.57 185.62,162.89
S$14846
  Bottom 0: 185.62,162.89 185.57,163.22
S$14847
  Bottom 0: 185.57,163.22 185.44,163.51
S$14848
  Bottom 0: 185.44,163.51 185.24,163.77
S$14849
  Bottom 0: 185.24,163.77 184.97,163.96
S$14850
  Bottom 0: 184.97,163.96 184.67,164.06
S$14851
  Bottom 0: 184.67,164.06 184.34,164.08
S$14852
  Bottom 0: 184.34,164.08 184.02,164.02
S$14853
  Bottom 0: 184.02,164.02 183.73,163.87
S$14854
  Bottom 0: 183.73,163.87 183.5,163.65
S$14855
  Bottom 0: 183.5,163.65 183.33,163.37
S$14856
  Bottom 0: 183.33,163.37 183.24,163.06
S$14857
  Bottom 0: 183.24,163.06 183.24,162.73
S$14858
  Bottom 0: 183.24,162.73 183.33,162.42
S$14859
  Bottom 0: 183.33,162.42 183.5,162.14
S$14860
  Bottom 0: 183.5,162.14 183.73,161.92
S$14861
  Bottom 0: 183.73,161.92 184.02,161.77
S$14862
  Bottom 0: 184.02,161.77 184.34,161.71
S$14863
  Bottom 0: 184.34,161.71 184.67,161.73
S$14864
  Bottom 0: 184.67,161.73 184.89,161.8
S$14865
  Bottom 0: 184.89,161.8 185.94,160.75
S$14866
  Bottom 0: 185.94,160.75 185.91,160.73
S$14867
  Bottom 0: 185.91,160.73 185.85,160.68
S$14868
  Bottom 0: 185.85,160.68 185.81,160.6
S$14869
  Bottom 0: 185.81,160.6 185.8,160.53
S$14870
  Bottom 0: 185.8,160.53 185.8,158.75
S$14871
  Bottom 0: 185.8,158.75 185.81,158.67
S$14872
  Bottom 0: 185.81,158.67 185.85,158.6
S$14873
  Bottom 0: 185.85,158.6 185.91,158.55
S$14874
  Bottom 0: 185.91,158.55 185.98,158.51
S$14875
  Bottom 0: 185.98,158.51 186.06,158.5
S$14876
  Bottom 0: 189.32,158.51 189.65,158.51
S$14877
  Bottom 0: 189.65,158.51 189.95,158.6
S$14878
  Bottom 0: 189.95,158.6 190.23,158.78
S$14879
  Bottom 0: 190.23,158.78 190.44,159.02
S$14880
  Bottom 0: 190.44,159.02 190.58,159.32
S$14881
  Bottom 0: 190.58,159.32 190.63,159.64
S$14882
  Bottom 0: 190.63,159.64 190.58,159.96
S$14883
  Bottom 0: 190.58,159.96 190.44,160.26
S$14884
  Bottom 0: 190.44,160.26 190.23,160.5
S$14885
  Bottom 0: 190.23,160.5 189.95,160.68
S$14886
  Bottom 0: 189.95,160.68 189.65,160.77
S$14887
  Bottom 0: 189.65,160.77 189.32,160.77
S$14888
  Bottom 0: 189.32,160.77 189.01,160.68
S$14889
  Bottom 0: 189.01,160.68 188.74,160.5
S$14890
  Bottom 0: 188.74,160.5 188.52,160.26
S$14891
  Bottom 0: 188.52,160.26 188.39,159.96
S$14892
  Bottom 0: 188.39,159.96 188.34,159.64
S$14893
  Bottom 0: 188.34,159.64 188.39,159.32
S$14894
  Bottom 0: 188.39,159.32 188.52,159.02
S$14895
  Bottom 0: 188.52,159.02 188.74,158.78
S$14896
  Bottom 0: 188.74,158.78 189.01,158.6
S$14897
  Bottom 0: 189.01,158.6 189.32,158.51
S$14898
  Bottom 0: 150.21,169.03 150.5,169.09
S$14899
  Bottom 0: 150.5,169.09 150.76,169.25
S$14900
  Bottom 0: 150.76,169.25 150.97,169.46
S$14901
  Bottom 0: 150.97,169.46 151.1,169.74
S$14902
  Bottom 0: 151.1,169.74 151.14,170.04
S$14903
  Bottom 0: 151.14,170.04 151.1,170.34
S$14904
  Bottom 0: 151.1,170.34 150.97,170.61
S$14905
  Bottom 0: 150.97,170.61 150.76,170.83
S$14906
  Bottom 0: 150.76,170.83 150.5,170.98
S$14907
  Bottom 0: 150.5,170.98 150.21,171.05
S$14908
  Bottom 0: 150.21,171.05 149.9,171.03
S$14909
  Bottom 0: 149.9,171.03 149.62,170.92
S$14910
  Bottom 0: 149.62,170.92 149.38,170.73
S$14911
  Bottom 0: 149.38,170.73 149.22,170.48
S$14912
  Bottom 0: 149.22,170.48 149.12,170.19
S$14913
  Bottom 0: 149.12,170.19 149.12,169.88
S$14914
  Bottom 0: 149.12,169.88 149.22,169.6
S$14915
  Bottom 0: 149.22,169.6 149.38,169.35
S$14916
  Bottom 0: 149.38,169.35 149.62,169.16
S$14917
  Bottom 0: 149.62,169.16 149.9,169.05
S$14918
  Bottom 0: 149.9,169.05 150.21,169.03
S$14919
  Bottom 0: 140.59,171.32 141.04,171.37
S$14920
  Bottom 0: 141.04,171.37 141.46,171.5
S$14921
  Bottom 0: 141.46,171.5 141.86,171.71
S$14922
  Bottom 0: 141.86,171.71 142.2,171.99
S$14923
  Bottom 0: 142.2,171.99 142.49,172.34
S$14924
  Bottom 0: 142.49,172.34 142.7,172.74
S$14925
  Bottom 0: 142.7,172.74 142.83,173.16
S$14926
  Bottom 0: 142.83,173.16 142.88,173.61
S$14927
  Bottom 0: 142.88,173.61 142.83,174.06
S$14928
  Bottom 0: 142.83,174.06 142.7,174.48
S$14929
  Bottom 0: 142.7,174.48 142.49,174.88
S$14930
  Bottom 0: 142.49,174.88 142.2,175.22
S$14931
  Bottom 0: 142.2,175.22 141.86,175.51
S$14932
  Bottom 0: 141.86,175.51 141.46,175.72
S$14933
  Bottom 0: 141.46,175.72 141.04,175.85
S$14934
  Bottom 0: 141.04,175.85 140.59,175.9
S$14935
  Bottom 0: 140.59,175.9 140.14,175.85
S$14936
  Bottom 0: 140.14,175.85 139.71,175.72
S$14937
  Bottom 0: 139.71,175.72 139.32,175.51
S$14938
  Bottom 0: 139.32,175.51 138.97,175.22
S$14939
  Bottom 0: 138.97,175.22 138.69,174.88
S$14940
  Bottom 0: 138.69,174.88 138.47,174.48
S$14941
  Bottom 0: 138.47,174.48 138.35,174.06
S$14942
  Bottom 0: 138.35,174.06 138.3,173.61
S$14943
  Bottom 0: 138.3,173.61 138.35,173.16
S$14944
  Bottom 0: 138.35,173.16 138.47,172.74
S$14945
  Bottom 0: 138.47,172.74 138.69,172.34
S$14946
  Bottom 0: 138.69,172.34 138.97,171.99
S$14947
  Bottom 0: 138.97,171.99 139.32,171.71
S$14948
  Bottom 0: 139.32,171.71 139.71,171.5
S$14949
  Bottom 0: 139.71,171.5 140.14,171.37
S$14950
  Bottom 0: 140.14,171.37 140.59,171.32
S$14951
  Bottom 0: 150.21,176.65 150.5,176.71
S$14952
  Bottom 0: 150.5,176.71 150.76,176.87
S$14953
  Bottom 0: 150.76,176.87 150.97,177.08
S$14954
  Bottom 0: 150.97,177.08 151.1,177.36
S$14955
  Bottom 0: 151.1,177.36 151.14,177.66
S$14956
  Bottom 0: 151.14,177.66 151.1,177.96
S$14957
  Bottom 0: 151.1,177.96 150.97,178.23
S$14958
  Bottom 0: 150.97,178.23 150.76,178.45
S$14959
  Bottom 0: 150.76,178.45 150.5,178.6
S$14960
  Bottom 0: 150.5,178.6 150.21,178.67
S$14961
  Bottom 0: 150.21,178.67 149.9,178.65
S$14962
  Bottom 0: 149.9,178.65 149.62,178.54
S$14963
  Bottom 0: 149.62,178.54 149.38,178.35
S$14964
  Bottom 0: 149.38,178.35 149.22,178.1
S$14965
  Bottom 0: 149.22,178.1 149.12,177.81
S$14966
  Bottom 0: 149.12,177.81 149.12,177.5
S$14967
  Bottom 0: 149.12,177.5 149.22,177.22
S$14968
  Bottom 0: 149.22,177.22 149.38,176.97
S$14969
  Bottom 0: 149.38,176.97 149.62,176.78
S$14970
  Bottom 0: 149.62,176.78 149.9,176.67
S$14971
  Bottom 0: 149.9,176.67 150.21,176.65
S$14972
  Bottom 0: 76.52,134.77 67.05,144.24
S$14973
  Bottom 0: 67.05,144.24 66.98,144.3
S$14974
  Bottom 0: 66.98,144.3 66.9,144.35
S$14975
  Bottom 0: 66.9,144.35 66.82,144.38
S$14976
  Bottom 0: 66.82,144.38 66.74,144.4
S$14977
  Bottom 0: 66.74,144.4 66.64,144.41
S$14978
  Bottom 0: 66.64,144.41 64.49,144.41
S$14979
  Bottom 0: 64.49,144.41 64.46,144.46
S$14980
  Bottom 0: 64.46,144.46 64.26,144.71
S$14981
  Bottom 0: 64.26,144.71 63.99,144.9
S$14982
  Bottom 0: 63.99,144.9 63.69,145.01
S$14983
  Bottom 0: 63.69,145.01 63.36,145.03
S$14984
  Bottom 0: 63.36,145.03 63.11,144.98
S$14985
  Bottom 0: 63.11,144.98 62.4,145.69
S$14986
  Bottom 0: 62.4,145.69 72.08,145.69
S$14987
  Bottom 0: 72.08,145.69 72.15,145.69
S$14988
  Bottom 0: 72.15,145.69 72.22,145.71
S$14989
  Bottom 0: 72.22,145.71 72.28,145.74
S$14990
  Bottom 0: 72.28,145.74 72.34,145.78
S$14991
  Bottom 0: 72.34,145.78 72.39,145.81
S$14992
  Bottom 0: 72.39,145.81 74.19,147.62
S$14993
  Bottom 0: 74.19,147.62 80.09,141.72
S$14994
  Bottom 0: 80.09,141.72 79.78,141.72
S$14995
  Bottom 0: 79.78,141.72 79.47,141.63
S$14996
  Bottom 0: 79.47,141.63 79.19,141.45
S$14997
  Bottom 0: 79.19,141.45 78.98,141.21
S$14998
  Bottom 0: 78.98,141.21 78.84,140.91
S$14999
  Bottom 0: 78.84,140.91 78.8,140.59
S$15000
  Bottom 0: 78.8,140.59 78.84,140.27
S$15001
  Bottom 0: 78.84,140.27 78.98,139.97
S$15002
  Bottom 0: 78.98,139.97 79.19,139.72
S$15003
  Bottom 0: 79.19,139.72 79.47,139.55
S$15004
  Bottom 0: 79.47,139.55 79.78,139.46
S$15005
  Bottom 0: 79.78,139.46 80.11,139.46
S$15006
  Bottom 0: 80.11,139.46 80.42,139.55
S$15007
  Bottom 0: 80.42,139.55 80.69,139.72
S$15008
  Bottom 0: 80.69,139.72 80.9,139.97
S$15009
  Bottom 0: 80.9,139.97 80.97,140.12
S$15010
  Bottom 0: 80.97,140.12 80.97,136.16
S$15011
  Bottom 0: 80.97,136.16 80.88,136.06
S$15012
  Bottom 0: 80.88,136.06 80.78,136.38
S$15013
  Bottom 0: 80.78,136.38 80.57,136.78
S$15014
  Bottom 0: 80.57,136.78 80.29,137.12
S$15015
  Bottom 0: 80.29,137.12 79.94,137.41
S$15016
  Bottom 0: 79.94,137.41 79.55,137.62
S$15017
  Bottom 0: 79.55,137.62 79.12,137.75
S$15018
  Bottom 0: 79.12,137.75 78.67,137.79
S$15019
  Bottom 0: 78.67,137.79 78.23,137.75
S$15020
  Bottom 0: 78.23,137.75 77.8,137.62
S$15021
  Bottom 0: 77.8,137.62 77.4,137.41
S$15022
  Bottom 0: 77.4,137.41 77.06,137.12
S$15023
  Bottom 0: 77.06,137.12 76.77,136.78
S$15024
  Bottom 0: 76.77,136.78 76.56,136.38
S$15025
  Bottom 0: 76.56,136.38 76.43,135.96
S$15026
  Bottom 0: 76.43,135.96 76.39,135.51
S$15027
  Bottom 0: 76.39,135.51 76.43,135.06
S$15028
  Bottom 0: 76.43,135.06 76.52,134.77
S$15029
  Bottom 0: 76.52,139.45 78.29,139.45
S$15030
  Bottom 0: 78.29,139.45 78.37,139.46
S$15031
  Bottom 0: 78.37,139.46 78.44,139.5
S$15032
  Bottom 0: 78.44,139.5 78.49,139.55
S$15033
  Bottom 0: 78.49,139.55 78.54,139.62
S$15034
  Bottom 0: 78.54,139.62 78.55,139.7
S$15035
  Bottom 0: 78.55,139.7 78.55,141.48
S$15036
  Bottom 0: 78.55,141.48 78.54,141.55
S$15037
  Bottom 0: 78.54,141.55 78.49,141.62
S$15038
  Bottom 0: 78.49,141.62 78.44,141.68
S$15039
  Bottom 0: 78.44,141.68 78.37,141.72
S$15040
  Bottom 0: 78.37,141.72 78.29,141.73
S$15041
  Bottom 0: 78.29,141.73 77.85,141.73
S$15042
  Bottom 0: 77.85,141.73 77.85,141.86
S$15043
  Bottom 0: 77.85,141.86 77.78,142.08
S$15044
  Bottom 0: 77.78,142.08 77.62,142.24
S$15045
  Bottom 0: 77.62,142.24 77.4,142.3
S$15046
  Bottom 0: 77.4,142.3 77.05,142.3
S$15047
  Bottom 0: 77.05,142.3 75.96,143.39
S$15048
  Bottom 0: 75.96,143.39 76.02,143.52
S$15049
  Bottom 0: 76.02,143.52 76.07,143.84
S$15050
  Bottom 0: 76.07,143.84 76.02,144.16
S$15051
  Bottom 0: 76.02,144.16 75.89,144.47
S$15052
  Bottom 0: 75.89,144.47 75.69,144.72
S$15053
  Bottom 0: 75.69,144.72 75.42,144.91
S$15054
  Bottom 0: 75.42,144.91 75.12,145.01
S$15055
  Bottom 0: 75.12,145.01 74.79,145.03
S$15056
  Bottom 0: 74.79,145.03 74.47,144.97
S$15057
  Bottom 0: 74.47,144.97 74.18,144.82
S$15058
  Bottom 0: 74.18,144.82 73.95,144.6
S$15059
  Bottom 0: 73.95,144.6 73.78,144.32
S$15060
  Bottom 0: 73.78,144.32 73.69,144.01
S$15061
  Bottom 0: 73.69,144.01 73.69,143.68
S$15062
  Bottom 0: 73.69,143.68 73.78,143.37
S$15063
  Bottom 0: 73.78,143.37 73.95,143.09
S$15064
  Bottom 0: 73.95,143.09 74.18,142.87
S$15065
  Bottom 0: 74.18,142.87 74.47,142.72
S$15066
  Bottom 0: 74.47,142.72 74.79,142.66
S$15067
  Bottom 0: 74.79,142.66 75.12,142.68
S$15068
  Bottom 0: 75.12,142.68 75.34,142.75
S$15069
  Bottom 0: 75.34,142.75 76.39,141.7
S$15070
  Bottom 0: 76.39,141.7 76.36,141.68
S$15071
  Bottom 0: 76.36,141.68 76.31,141.62
S$15072
  Bottom 0: 76.31,141.62 76.27,141.55
S$15073
  Bottom 0: 76.27,141.55 76.26,141.48
S$15074
  Bottom 0: 76.26,141.48 76.26,139.7
S$15075
  Bottom 0: 76.26,139.7 76.27,139.62
S$15076
  Bottom 0: 76.27,139.62 76.31,139.55
S$15077
  Bottom 0: 76.31,139.55 76.36,139.5
S$15078
  Bottom 0: 76.36,139.5 76.44,139.46
S$15079
  Bottom 0: 76.44,139.46 76.52,139.45
S$15080
  Bottom 0: 81.92,136.11 81.85,136.16
S$15081
  Bottom 0: 81.85,136.16 81.85,141.03
S$15082
  Bottom 0: 81.85,141.03 81.85,141.1
S$15083
  Bottom 0: 81.85,141.1 81.83,141.17
S$15084
  Bottom 0: 81.83,141.17 81.81,141.23
S$15085
  Bottom 0: 81.81,141.23 81.77,141.29
S$15086
  Bottom 0: 81.77,141.29 81.73,141.35
S$15087
  Bottom 0: 81.73,141.35 74.71,148.37
S$15088
  Bottom 0: 74.71,148.37 77.1,150.77
S$15089
  Bottom 0: 77.1,150.77 77.13,150.75
S$15090
  Bottom 0: 77.13,150.75 77.46,150.65
S$15091
  Bottom 0: 77.46,150.65 77.81,150.63
S$15092
  Bottom 0: 77.81,150.63 78.16,150.69
S$15093
  Bottom 0: 78.16,150.69 78.47,150.84
S$15094
  Bottom 0: 78.47,150.84 78.74,151.06
S$15095
  Bottom 0: 78.74,151.06 78.95,151.35
S$15096
  Bottom 0: 78.95,151.35 79.08,151.67
S$15097
  Bottom 0: 79.08,151.67 79.12,152.02
S$15098
  Bottom 0: 79.12,152.02 79.11,152.14
S$15099
  Bottom 0: 79.11,152.14 83.4,147.85
S$15100
  Bottom 0: 83.4,147.85 83.4,144.6
S$15101
  Bottom 0: 83.4,144.6 83.31,144.72
S$15102
  Bottom 0: 83.31,144.72 83.04,144.91
S$15103
  Bottom 0: 83.04,144.91 82.74,145.01
S$15104
  Bottom 0: 82.74,145.01 82.41,145.03
S$15105
  Bottom 0: 82.41,145.03 82.09,144.97
S$15106
  Bottom 0: 82.09,144.97 81.8,144.82
S$15107
  Bottom 0: 81.8,144.82 81.57,144.6
S$15108
  Bottom 0: 81.57,144.6 81.4,144.32
S$15109
  Bottom 0: 81.4,144.32 81.31,144.01
S$15110
  Bottom 0: 81.31,144.01 81.31,143.68
S$15111
  Bottom 0: 81.31,143.68 81.4,143.37
S$15112
  Bottom 0: 81.4,143.37 81.57,143.09
S$15113
  Bottom 0: 81.57,143.09 81.8,142.87
S$15114
  Bottom 0: 81.8,142.87 81.92,142.81
S$15115
  Bottom 0: 81.92,142.81 81.92,136.11
S$15116
  Bottom 0: 49.17,139.18 46.58,141.76
S$15117
  Bottom 0: 46.58,141.76 46.58,143.8
S$15118
  Bottom 0: 46.58,143.8 46.65,143.85
S$15119
  Bottom 0: 46.65,143.85 46.78,144.06
S$15120
  Bottom 0: 46.78,144.06 46.83,144.31
S$15121
  Bottom 0: 46.83,144.31 46.78,144.56
S$15122
  Bottom 0: 46.78,144.56 46.66,144.76
S$15123
  Bottom 0: 46.66,144.76 55.08,144.76
S$15124
  Bottom 0: 55.08,144.76 54.9,144.59
S$15125
  Bottom 0: 54.9,144.59 54.73,144.32
S$15126
  Bottom 0: 54.73,144.32 54.64,144
S$15127
  Bottom 0: 54.64,144 54.64,143.68
S$15128
  Bottom 0: 54.64,143.68 54.73,143.36
S$15129
  Bottom 0: 54.73,143.36 54.9,143.09
S$15130
  Bottom 0: 54.9,143.09 55.13,142.87
S$15131
  Bottom 0: 55.13,142.87 55.42,142.72
S$15132
  Bottom 0: 55.42,142.72 55.74,142.65
S$15133
  Bottom 0: 55.74,142.65 56.07,142.67
S$15134
  Bottom 0: 56.07,142.67 56.29,142.75
S$15135
  Bottom 0: 56.29,142.75 57.34,141.69
S$15136
  Bottom 0: 57.34,141.69 57.32,141.68
S$15137
  Bottom 0: 57.32,141.68 57.27,141.62
S$15138
  Bottom 0: 57.27,141.62 57.22,141.55
S$15139
  Bottom 0: 57.22,141.55 57.22,141.48
S$15140
  Bottom 0: 57.22,141.48 57.22,139.69
S$15141
  Bottom 0: 57.22,139.69 51.1,139.69
S$15142
  Bottom 0: 51.1,139.69 51.07,139.85
S$15143
  Bottom 0: 51.07,139.85 50.94,140.13
S$15144
  Bottom 0: 50.94,140.13 50.74,140.34
S$15145
  Bottom 0: 50.74,140.34 50.48,140.5
S$15146
  Bottom 0: 50.48,140.5 50.18,140.56
S$15147
  Bottom 0: 50.18,140.56 49.88,140.54
S$15148
  Bottom 0: 49.88,140.54 49.6,140.43
S$15149
  Bottom 0: 49.6,140.43 49.36,140.24
S$15150
  Bottom 0: 49.36,140.24 49.19,140
S$15151
  Bottom 0: 49.19,140 49.1,139.71
S$15152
